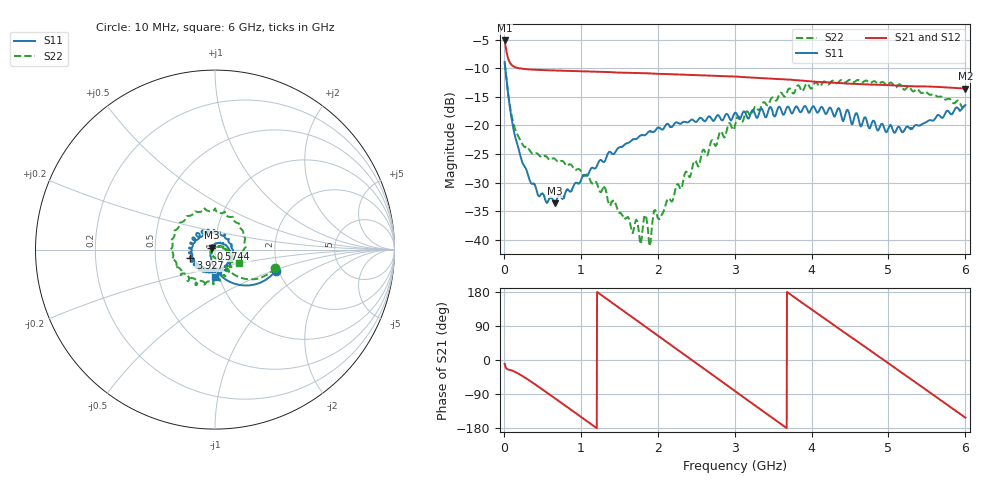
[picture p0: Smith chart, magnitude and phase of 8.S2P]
!Agilent Technologies,E5071C,MY46316741,A.11.02
!Date: Tue Oct 20 14:45:01 2020
!Data & Calibration Information:
!Freq	S11:SOLT4(ON)	S21:SOLT4(ON)	S12:SOLT4(ON)	S22:SOLT4(ON)
!PortZ  Port1:50+j0  Port2:50+j0
!Above PortZ is port z conversion or system Z0 setting when saving the data.
!When reading, reference impedance value at option line is always used.
# Hz S dB R 50
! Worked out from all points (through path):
!   1561 points, 10 MHz to 6 GHz, reference 50 ohm
!   highest |S21| = -5.13 dB at 10 MHz (marker M1); lowest = -13.6 dB at 6 GHz (marker M2)
!   group delay of S21, straight-line fit = 401 ps
!   lowest |S11| = -33.6 dB at 662.8 MHz (marker M3), VSWR 1.04, Z = 48.3 + j1.12 ohm
!   |S11| at or under -10 dB: 20.19 MHz to end of sweep
!   |S22| runs from -41.1 to -9.1 dB; largest |S21 - S12| = 0.0052
!   S11 on the Smith chart (normalised r, x): 10 MHz: 1.93, -0.52; 574.4 MHz: 0.96, +0.01; 3.927 GHz: 0.75, -0.07; 6 GHz: 0.96, -0.29
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1e7  -8.88 -19.2  -5.13 -10.2  -5.22 -10.1  -9.07 -16.7
7.911538e7  -16.90 -78.6  -9.03 -26.3  -9.06 -26.3  -16.59 -55.4
2.288654e8  -25.98 -115.9  -10.08 -40.7  -10.11 -40.6  -22.97 -56.4
5.744423e8  -33.25 163.5  -10.35 -88.1  -10.38 -88.1  -25.78 -70.2
6.627564e8  -33.63 146.3  -10.39 -100.8  -10.41 -100.9  -25.83 -77.4
1.012173e9  -29.26 81.0  -10.52 -151.4  -10.55 -151.6  -28.32 -107.3
1.350071e9  -24.96 38.9  -10.65 159.3  -10.68 159.1  -33.07 -142.3
1.726365e9  -22.35 2.5  -10.83 104.6  -10.86 104.5  -36.58 141.9
1.776282e9  -21.74 -2.8  -10.85 97.4  -10.87 97.1  -40.63 128.8
1.833878e9  -21.71 -7.6  -10.86 88.9  -10.90 88.8  -35.80 110.0
1.895314e9  -21.03 -13.2  -10.89 79.9  -10.92 79.7  -41.13 98.6
1.95675e9  -21.09 -20.1  -10.94 70.8  -10.97 70.7  -35.03 80.0
2.006667e9  -20.34 -23.2  -10.97 63.6  -10.99 63.5  -36.29 83.2
2.486635e9  -19.36 -61.8  -11.19 -6.2  -11.22 -6.5  -26.15 21.0
3.005e9  -17.79 -98.1  -11.45 -82.1  -11.49 -82.3  -20.01 -37.0
3.508006e9  -18.18 -126.4  -11.83 -155.3  -11.87 -155.4  -15.23 -80.2
3.926538e9  -16.74 -161.5  -12.23 144.0  -12.26 143.8  -12.82 -132.5
4.007173e9  -16.80 -174.0  -12.31 132.6  -12.33 132.5  -13.46 -140.4
4.441064e9  -17.98 134.9  -12.66 70.6  -12.67 70.4  -12.49 173.7
5.001667e9  -20.41 56.7  -12.95 -9.2  -12.97 -9.2  -12.75 106.1
5.516192e9  -19.20 -27.8  -13.19 -82.6  -13.20 -82.7  -14.46 44.4
6e9  -16.45 -89.7  -13.55 -152.2  -13.56 -152.2  -16.27 -29.0
